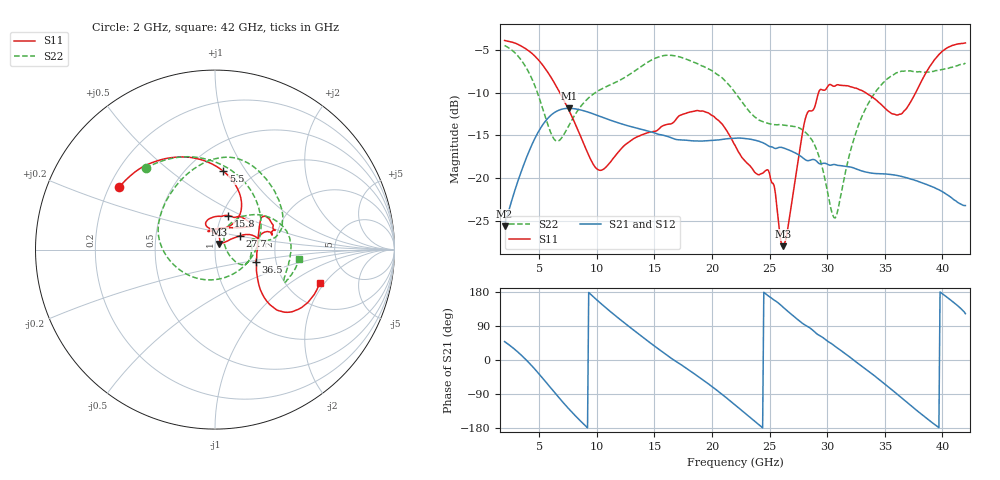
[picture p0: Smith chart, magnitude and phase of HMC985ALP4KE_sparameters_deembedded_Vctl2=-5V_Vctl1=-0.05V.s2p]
!s2p File: Measurements: S11, S21, S12, S22
# GHz S dB R 50.0
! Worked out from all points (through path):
!   401 points, 2 GHz to 42 GHz, reference 50 ohm
!   highest |S21| = -11.83 dB at 7.6 GHz (marker M1); lowest = -25.6 dB at 2 GHz (marker M2)
!   lowest |S11| = -27.9 dB at 26.2 GHz (marker M3), VSWR 1.08, Z = 52.5 + j3.31 ohm
!   |S11| at or under -10 dB: 6.79 GHz to 29.26 GHz (22.47 GHz wide, 125 % of centre); 33.32 GHz to 37.69 GHz (4.368 GHz wide, 12.3 % of centre)
!   |S22| runs from -24.6 to -4.5 dB; largest |S21 - S12| = 0.00022
!   S11 on the Smith chart (normalised r, x): 2 GHz: 0.24, +0.28; 5.5 GHz: 0.73, +0.79; 15.8 GHz: 1.07, +0.42; 27.7 GHz: 1.30, +0.21; 36.5 GHz: 1.57, -0.22; 42 GHz: 3.02, -1.82
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2  -3.92 147.1  -25.58 48.6  -25.59 48.6  -4.51 130.5
3.6  -4.70 120.4  -18.63 8.4  -18.64 8.4  -6.52 85.0
5.5  -7.15 83.9  -13.41 -55.2  -13.41 -55.2  -12.69 2.5
6.5  -9.29 66.7  -12.19 -91.8  -12.19 -91.8  -15.64 -69.0
7.6  -12.11 55.2  -11.83 -129.8  -11.84 -129.8  -13.79 -135.8
8.7  -15.43 55.9  -12.06 -164.3  -12.06 -164.3  -11.46 -170.2
10.4  -19.05 90.2  -12.83 148.0  -12.83 148.0  -9.59 162.6
12.7  -15.86 108.1  -13.87 90.7  -13.88 90.7  -8.02 129.1
15.4  -14.23 75.9  -14.88 28.2  -14.89 28.2  -5.83 87.6
15.8  -13.84 69.1  -14.98 19.3  -14.99 19.3  -5.69 82.5
19.4  -12.25 33.7  -15.64 -56.5  -15.64 -56.5  -7.04 35.7
22  -16.15 51.6  -15.31 -118.4  -15.31 -118.4  -9.99 10.3
24.9  -19.07 104.5  -16.22 169.0  -16.23 169.0  -13.61 13.4
26.2  -27.91 51.5  -16.45 138.5  -16.46 138.5  -13.79 -1.3
27.7  -16.02 29.3  -17.41 100.5  -17.41 100.5  -14.22 -21.6
28.7  -12.12 13.2  -17.81 80.0  -17.82 80.0  -15.56 -29.9
30.7  -9.23 21.2  -18.40 35.8  -18.41 35.8  -24.61 21.9
32.8  -9.66 34.3  -19.04 -11.9  -19.05 -11.8  -13.50 54.3
35.4  -12.24 11.6  -19.53 -73.1  -19.54 -73.1  -8.23 22.2
36.5  -12.44 -16.4  -19.79 -100.9  -19.80 -100.8  -7.50 8.2
39.5  -5.90 -42.8  -21.21 -173.9  -21.21 -173.9  -7.43 -24.9
42  -4.21 -17.7  -23.17 122.2  -23.19 122.3  -6.55 -6.2
